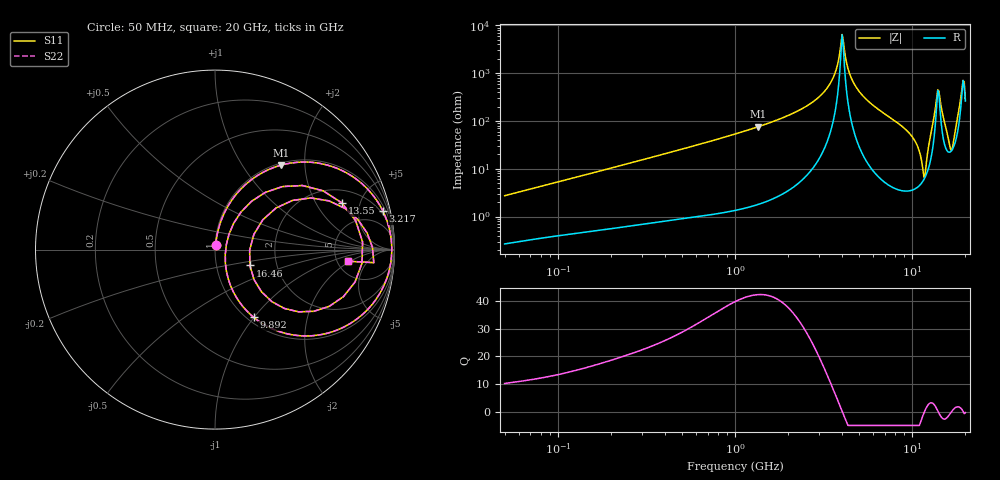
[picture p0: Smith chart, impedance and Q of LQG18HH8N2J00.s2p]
!Murata Part Number: LQG18HH8N2J00
!These Parameters are Measured in Series Mode Connection
!  o--[Z]--o
!Port1  Port2
!  o-------o
!Freq. Start=50[MHz] Stop=20[GHz], 401[Steps]
# Hz S RI R 50
!Freq.(Hz) S11(Real) S11(Imag) S21(Real) S21(Imag) S12(Real) S12(Imag) S22(Real) S22(Imag)
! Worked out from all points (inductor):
!   401 points, 50 MHz to 20 GHz, reference 50 ohm
!   read as one part in series: L = 8.57 nH near 51.52 MHz
!   highest Q = 42.2 at 1.349 GHz (marker M1), where L = 8.94 nH
!   self-resonance near 4.027 GHz
!   S11 on the Smith chart (normalised r, x): 50 MHz: 1.01, +0.05; 3.217 GHz: 1.56, +8.50; 9.892 GHz: 1.07, -0.99; 13.55 GHz: 2.81, +3.38; 16.46 GHz: 1.45, -0.27; 20 GHz: 6.24, -1.79
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5e7  0.00341 0.0271  0.9966 -0.0271  0.9966 -0.0271  0.00341 0.0271
1.364002e8  0.0096 0.0704  0.9904 -0.0704  0.9904 -0.0704  0.0096 0.0704
3.721004e8  0.0421 0.1817  0.9579 -0.1817  0.9579 -0.1817  0.0421 0.1817
1e9  0.2275 0.4068  0.7725 -0.4068  0.7725 -0.4068  0.2275 0.4068
1.349283e9  0.3679 0.4705  0.6321 -0.4705  0.6321 -0.4705  0.3679 0.4705
2.728004e9  0.8479 0.3395  0.1521 -0.3395  0.1521 -0.3395  0.8479 0.3395
3.216634e9  0.9351 0.2156  0.0649 -0.2156  0.0649 -0.2156  0.9351 0.2156
3.626126e9  0.9734 0.1062  0.0266 -0.1062  0.0266 -0.1062  0.9734 0.1062
4.026975e9  0.9849 0.00207  0.0151 -0.00207  0.0151 -0.00207  0.9849 0.00207
4.405649e9  0.9764 -0.0896  0.0236 0.0896  0.0236 0.0896  0.9764 -0.0896
4.89267e9  0.9439 -0.1942  0.0561 0.1942  0.0561 0.1942  0.9439 -0.1942
7.442007e9  0.5909 -0.4736  0.4091 0.4736  0.4091 0.4736  0.5909 -0.4736
9.892087e9  0.2151 -0.377  0.7849 0.377  0.7849 0.377  0.2151 -0.377
1.166392e10  0.0572 -0.0262  0.9428 0.0262  0.9428 0.0262  0.0572 -0.0262
1.276073e10  0.2804 0.3188  0.7196 -0.3188  0.7196 -0.3188  0.2804 0.3188
1.354865e10  0.7061 0.2607  0.2939 -0.2607  0.2939 -0.2607  0.7061 0.2607
1.417136e10  0.8192 -0.0758  0.1808 0.0758  0.1808 0.0758  0.8192 -0.0758
1.504638e10  0.5505 -0.3438  0.4495 0.3438  0.4495 0.3438  0.5505 -0.3438
1.646126e10  0.1944 -0.0883  0.8056 0.0883  0.8056 0.0883  0.1944 -0.0883
1.800918e10  0.5339 0.2878  0.4661 -0.2878  0.4661 -0.2878  0.5339 0.2878
1.912117e10  0.8472 0.0929  0.1528 -0.0929  0.1528 -0.0929  0.8472 0.0929
2e10  0.7397 -0.0645  0.2603 0.0645  0.2603 0.0645  0.7397 -0.0645
